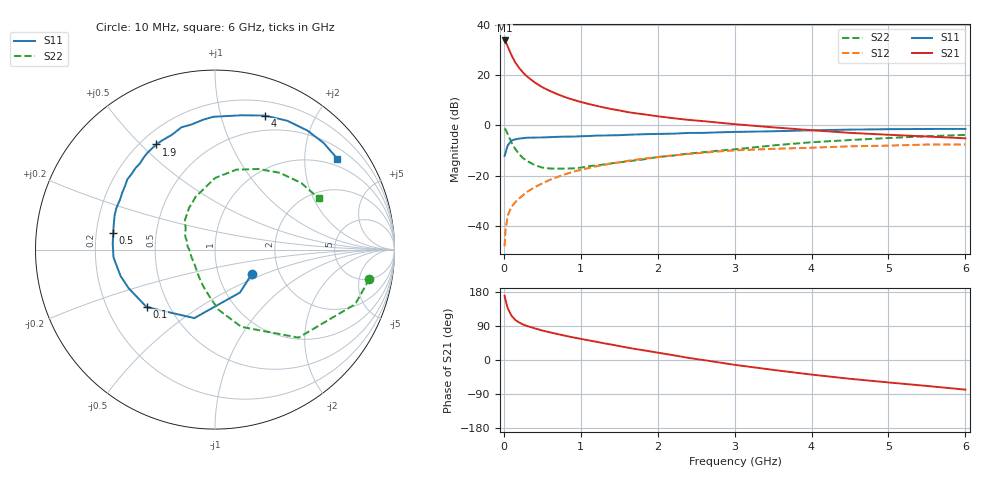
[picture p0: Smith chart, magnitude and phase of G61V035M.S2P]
! SIEMENS Small Signal Semiconductors
! BFG193
! Si NPN RF Bipolar Junction Transistor in SOT223
! VCE = 1 V  IC = 35 mA
! Common Emitter S-Parameters:  August  1996
# GHz  S  MA  R  50
!  f  S11  S21  S12  S22
! GHz  MAG  ANG  MAG  ANG  MAG  ANG  MAG  ANG
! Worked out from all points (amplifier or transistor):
!   36 points, 10 MHz to 6 GHz, reference 50 ohm
!   highest |S21| = 33.9 dB at 10 MHz (marker M1)
!   |S21| within 3 dB of that: start of sweep to 58.88 MHz
!   unconditionally stable (mu >= 1): 396.5 MHz to 3.687 GHz
!   at 250 MHz: K = 0.91, MSG = 24.4 dB, |S12| = -27.9 dB
!   at 1.4 GHz: K = 1.07, MAG = 9.2 dB, |S12| = -15.2 dB
!   at 6 GHz: K = 0.98, MSG = 1.2 dB, |S12| = -7.6 dB
!   S11 on the Smith chart (normalised r, x): 10 MHz: 1.45, -0.41; 100 MHz: 0.37, -0.32; 500 MHz: 0.27, +0.08; 1.9 GHz: 0.26, +0.56; 4 GHz: 0.34, +1.39; 6 GHz: 0.78, +2.83
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0.01  0.2459 -33.2  49.38 169.4  0.0039 83.2  0.8755 -10.7
0.02  0.2767 -59.8  47.03 160.2  0.0075 75.0  0.8383 -21.3
0.05  0.3988 -106.8  37.59 136.8  0.0159 62.6  0.6761 -46.5
0.1  0.4978 -140.0  24.99 116.8  0.0238 57.2  0.4545 -71.2
0.15  0.5273 -156.0  17.87 105.4  0.0295 56.9  0.3361 -86.6
0.2  0.5457 -164.2  13.9 98.9  0.035 59.0  0.2666 -96.1
0.25  0.5554 -170.7  11.28 93.7  0.0405 60.6  0.2216 -105.9
0.3  0.5671 -175.7  9.496 89.8  0.047 62.1  0.1963 -113.2
0.4  0.5707 176.8  7.203 83.7  0.0584 62.5  0.1618 -127.6
0.5  0.5749 170.6  5.78 77.8  0.0697 62.1  0.1441 -139.5
0.6  0.5818 165.7  4.849 73.0  0.0823 61.5  0.1378 -148.8
0.8  0.5966 157.0  3.642 63.9  0.1061 58.2  0.1378 -167.1
1.1  0.613 145.1  2.676 51.9  0.1407 53.0  0.1529 174.1
1.5  0.637 131.0  1.989 36.8  0.1836 43.7  0.1833 155.1
1.9  0.6709 119.2  1.597 22.8  0.2242 34.4  0.2206 139.5
2.2  0.6835 110.5  1.392 12.7  0.2521 26.9  0.2494 129.2
2.8  0.7271 95.1  1.131 -6.5  0.3032 12.2  0.3142 110.0
3.5  0.763 78.8  0.913 -26.1  0.3408 -5.6  0.3987 90.0
4  0.7972 69.5  0.801 -38.5  0.3584 -15.3  0.4608 75.1
4.5  0.8232 60.7  0.709 -49.6  0.3824 -25.0  0.5104 61.6
5.5  0.8482 44.5  0.6 -68.5  0.415 -47.4  0.6073 37.7
6  0.8491 36.6  0.552 -78.2  0.4145 -60.0  0.6452 26.2
